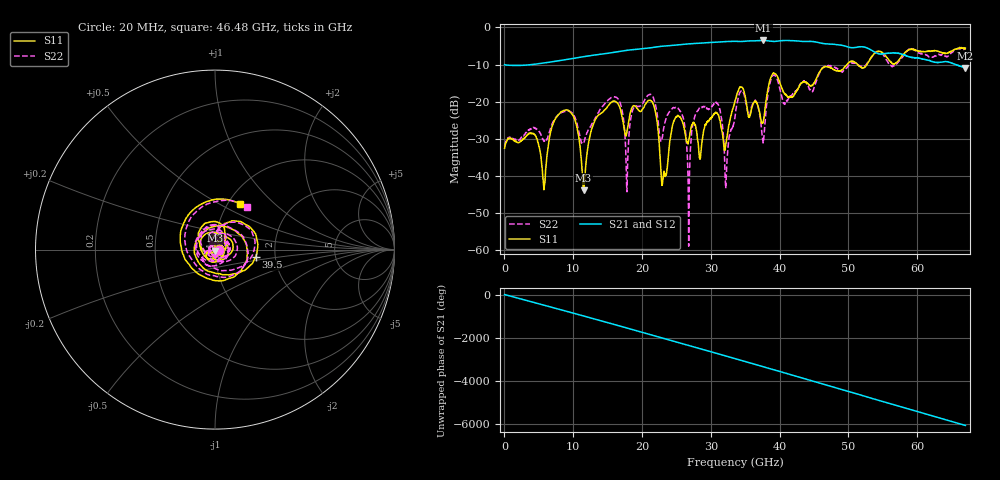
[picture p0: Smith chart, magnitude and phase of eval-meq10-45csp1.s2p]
!Keysight Technologies,N5247B,US58420632,A.14.00.23
!Date: Monday, March 14, 2022 13:47:07
!Correction: S22(C  2-Port  )
!S42(C  2-Port  )
!S24(C  2-Port  )
!S44(C  2-Port  )
!S2P File: Measurement: :
# Hz S  dB  R 50
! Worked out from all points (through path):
!   3350 points, 20 MHz to 67 GHz, reference 50 ohm
!   highest |S21| = -3.50 dB at 37.64 GHz (marker M1); lowest = -10.9 dB at 67 GHz (marker M2)
!   lowest |S11| = -44.0 dB at 11.5 GHz (marker M3), VSWR 1.01, Z = 50 - j0.631 ohm
!   |S11| at or under -10 dB: start of sweep to 49.8 GHz; 51.35 GHz to 52.69 GHz (1.342 GHz wide, 2.58 % of centre)
!   |S22| runs from -59.0 to -5.6 dB; largest |S21 - S12| = 0.0036
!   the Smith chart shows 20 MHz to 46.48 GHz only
!   S11 on the Smith chart (normalised r, x): 20 MHz: 1.05, +0.00; 39.5 GHz: 1.58, -0.14; 46.48 GHz: 1.14, +0.64
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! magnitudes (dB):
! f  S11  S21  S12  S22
! 20 MHz  -32.6  -10.0  -10.1  -32.0
! 5.76 GHz  -43.4  -9.6  -9.6  -30.7
! 9.12 GHz  -22.2  -8.6  -8.6  -22.5
! 11.2 GHz  -36.3  -8.0  -8.0  -31.2
! 11.5 GHz  -44.0  -7.9  -7.9  -31.1
! 15.66 GHz  -20.1  -6.8  -6.8  -18.8
! 17.8 GHz  -28.2  -6.2  -6.2  -44.3
! 18.92 GHz  -21.1  -6.0  -6.0  -21.5
! 22.36 GHz  -28.4  -5.2  -5.2  -25.8
! 23.14 GHz  -39.2  -5.0  -5.0  -27.2
! 25.46 GHz  -24.2  -4.7  -4.7  -22.5
! 26.78 GHz  -30.4  -4.4  -4.4  -59.0
! 28.16 GHz  -31.2  -4.3  -4.3  -22.4
! 31.04 GHz  -23.6  -3.9  -3.9  -20.7
! 32.22 GHz  -31.1  -3.8  -3.8  -41.2
! 33.52 GHz  -19.8  -3.7  -3.8  -24.1
! 37.64 GHz  -25.1  -3.5  -3.5  -30.9
! 39.5 GHz  -12.8  -3.7  -3.7  -13.4
! 44.68 GHz  -15.6  -3.8  -3.8  -17.1
! 46.48 GHz  -10.7  -4.4  -4.4  -10.6
! 55.84 GHz  -8.7  -7.0  -6.9  -9.7
! 67 GHz  -5.6  -10.9  -10.9  -5.7
